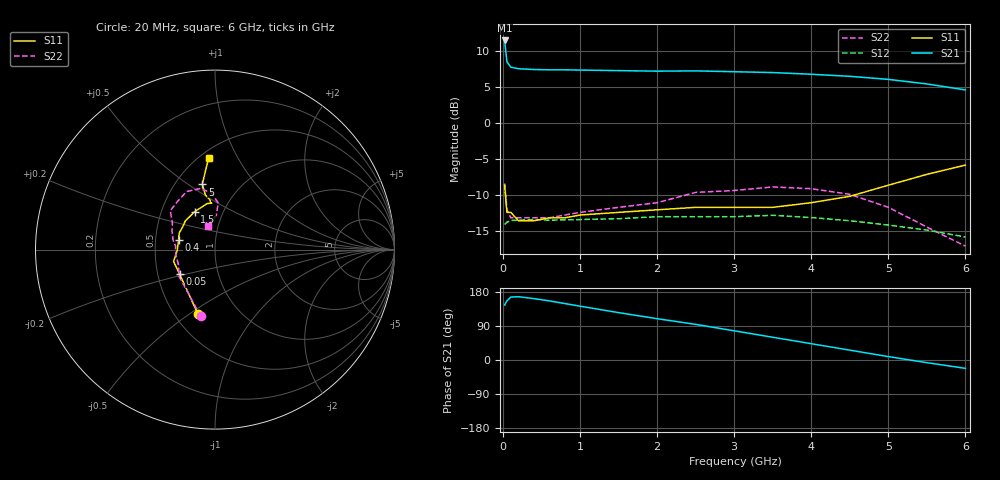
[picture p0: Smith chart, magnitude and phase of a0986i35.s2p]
!  MSA-0986 S AND NOISE PARAMETERS
!  Id=35mA  LAST UPDATED 07-27-92
# ghz s ma r 50
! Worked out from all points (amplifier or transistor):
!   18 points, 20 MHz to 6 GHz, reference 50 ohm
!   highest |S21| = 11.4 dB at 20 MHz (marker M1)
!   |S21| within 3 dB of that: start of sweep to 53.59 MHz
!   unconditionally stable (mu >= 1): 40.77 MHz to end of sweep
!   at 200 MHz: K = 1.20, MAG = 7.8 dB, |S12| = -13.5 dB
!   at 2 GHz: K = 1.16, MAG = 7.6 dB, |S12| = -13.0 dB
!   at 6 GHz: K = 1.47, MAG = 6.1 dB, |S12| = -15.8 dB
!   lowest NFmin = 6.00 dB at 100 MHz
!   S11 on the Smith chart (normalised r, x): 20 MHz: 0.65, -0.54; 50 MHz: 0.65, -0.19; 400 MHz: 0.66, +0.07; 1.5 GHz: 0.73, +0.33; 5 GHz: 0.68, +0.57; 6 GHz: 0.56, +0.76
0.02  0.37 -105.0  3.72 145.0  0.198 18.0  0.38 -102.0
0.05  0.24 -145.0  2.65 156.0  0.205 5.0  0.25 -143.0
0.1  0.24 -164.0  2.43 166.0  0.211 4.0  0.22 -158.0
0.2  0.21 -179.0  2.37 167.0  0.212 1.0  0.22 -172.0
0.4  0.21 165.0  2.34 162.0  0.214 -1.0  0.22 179.0
0.6  0.22 155.0  2.33 156.0  0.212 -2.0  0.22 175.0
0.8  0.22 145.0  2.33 149.0  0.213 -2.0  0.23 171.0
1  0.23 136.0  2.32 142.0  0.214 -4.0  0.24 167.0
1.5  0.24 118.0  2.3 125.0  0.217 -6.0  0.26 157.0
2  0.25 106.0  2.28 109.0  0.224 -10.0  0.28 148.0
2.5  0.26 100.0  2.29 94.0  0.224 -12.0  0.33 139.0
3  0.26 94.0  2.26 77.0  0.224 -15.0  0.34 128.0
3.5  0.26 95.0  2.23 60.0  0.229 -21.0  0.36 116.0
4  0.28 96.0  2.17 43.0  0.221 -25.0  0.35 104.0
4.5  0.31 100.0  2.1 26.0  0.21 -31.0  0.32 94.0
5  0.37 101.0  2 9.0  0.196 -35.0  0.26 86.0
5.5  0.44 97.0  1.86 -7.0  0.181 -38.0  0.19 88.0
6  0.51 94.0  1.69 -22.0  0.162 -37.0  0.14 107.0
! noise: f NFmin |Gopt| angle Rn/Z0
0.1  6  0.11  22  1.02
0.5  6  0.09  -3  1.03
1  6  0.09  -17  1.03
2  6.1  0.1  -52  1.07
3  6.2  0.16  -70  1.16
4  6.2  0.24  -74  1.37
